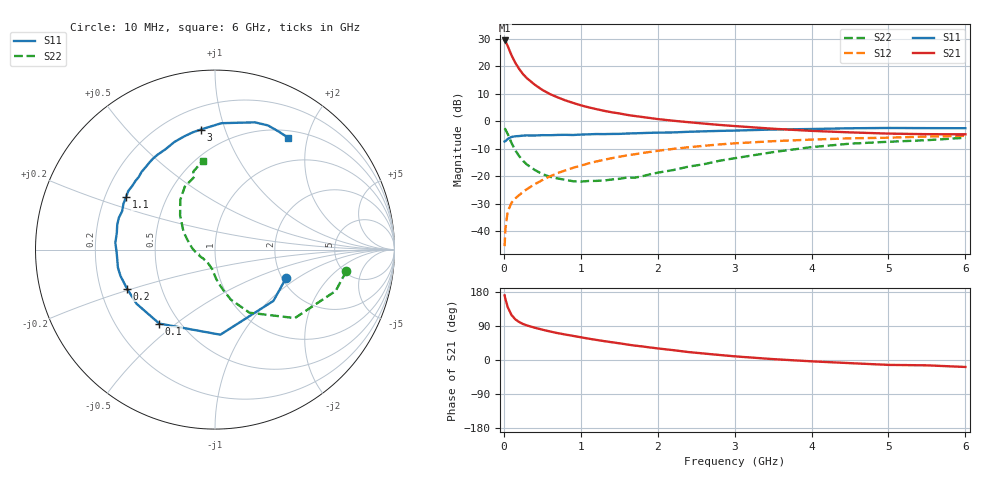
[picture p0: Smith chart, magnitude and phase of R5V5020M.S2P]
! SIEMENS Small Signal Semiconductors
! BFR183
! Si NPN RF Bipolar Junction Transistor in SOT23
! VCE = 0.5 V  IC = 20 mA
! Common Emitter S-Parameters:  May  1996
# GHz  S  MA  R  50
!  f  S11  S21  S12  S22
! GHz  MAG  ANG  MAG  ANG  MAG  ANG  MAG  ANG
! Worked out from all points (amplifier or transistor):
!   36 points, 10 MHz to 6 GHz, reference 50 ohm
!   highest |S21| = 29.4 dB at 10 MHz (marker M1)
!   |S21| within 3 dB of that: start of sweep to 64.65 MHz
!   unconditionally stable (mu >= 1): start of sweep to 12.55 MHz; 236.9 MHz to end of sweep
!   at 250 MHz: K = 1.02, MAG = 20.5 dB, |S12| = -25.8 dB
!   at 1.4 GHz: K = 1.24, MAG = 5.5 dB, |S12| = -13.5 dB
!   at 6 GHz: K = 1.06, MAG = -1.3 dB, |S12| = -5.3 dB
!   S11 on the Smith chart (normalised r, x): 10 MHz: 2.11, -0.81; 100 MHz: 0.39, -0.44; 200 MHz: 0.31, -0.19; 1.1 GHz: 0.29, +0.25; 3 GHz: 0.34, +0.83; 6 GHz: 0.60, +1.68
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0.01  0.4268 -21.5  29.48 170.5  0.0053 79.4  0.7416 -9.3
0.02  0.4331 -41.3  28.46 161.4  0.0108 73.4  0.7107 -18.9
0.05  0.4751 -86.4  23.42 139.7  0.0226 61.4  0.5862 -40.6
0.1  0.516 -127.0  15.8 118.5  0.0329 53.7  0.4004 -61.4
0.15  0.5311 -145.4  11.47 107.2  0.0394 52.7  0.2921 -72.4
0.2  0.5363 -156.1  8.895 100.1  0.0452 55.1  0.2311 -78.3
0.25  0.5468 -164.5  7.164 94.9  0.0514 56.9  0.1892 -83.8
0.3  0.55 -169.5  6.057 91.2  0.0579 58.9  0.1624 -87.8
0.4  0.548 -178.1  4.637 85.3  0.0709 61.2  0.13 -93.2
0.5  0.5565 176.1  3.714 80.1  0.0845 62.7  0.1087 -98.7
0.6  0.5549 170.3  3.114 75.3  0.0988 63.1  0.0971 -105.5
0.7  0.5618 165.9  2.711 70.9  0.1134 63.1  0.0906 -111.2
0.9  0.5599 157.6  2.15 63.6  0.1413 62.1  0.0806 -120.6
1.1  0.5755 149.5  1.788 56.4  0.17 60.1  0.0815 -132.2
1.3  0.5815 142.9  1.546 49.9  0.1981 57.7  0.0829 -144.7
1.6  0.5959 133.3  1.302 41.0  0.2379 53.5  0.0941 -159.6
2.2  0.6238 116.1  1.019 26.0  0.3125 44.3  0.1287 175.5
3  0.6737 96.7  0.815 9.7  0.3952 31.2  0.2114 147.6
3.5  0.7052 87.1  0.728 2.3  0.4322 23.3  0.273 135.4
4.5  0.743 72.6  0.625 -8.3  0.4877 9.3  0.3892 115.6
5.5  0.7473 61.5  0.58 -14.1  0.5258 -1.4  0.4505 105.6
6  0.7447 56.9  0.576 -18.4  0.5403 -8.4  0.4991 97.9
